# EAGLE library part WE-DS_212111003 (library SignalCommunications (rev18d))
WE-DS D-SUB-Filter, Solder Pin Straight Characteristics Standard type filtered with 1000 pF High attenuation: max. ≥ 40 dB @ 180 MHz Choice of UNC 4/40 or through hole Rated voltage: 100 VDC Rated current @ 20 ºC: 5 A Withstand voltage: 250 VRMS Insulation resistance: min. 1000 MΩ Operating temperature: –55 ºC to +125 ºC Applications Filtering of interfaces External connection to -printer -sensor -display Details see: http://katalog.we-online.de/en/pbs/Filter_gerade Created on 2015-05-04 2015 (C) Wurth Elektronik
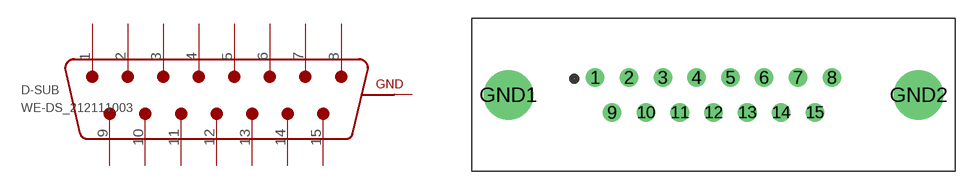
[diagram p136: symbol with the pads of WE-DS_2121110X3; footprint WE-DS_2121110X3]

Designator prefix D-SUB

## WE-DS_212111003 (WE-NUMBER: 212111003/15pins_male)  [WE-DS_2121110X3]
1  1  pas
2  2  pas
3  3  pas
4  4  pas
5  5  pas
6  6  pas
7  7  pas
8  8  pas
9  9  pas
10  10  pas
11  11  pas
12  12  pas
13  13  pas
14  14  pas
15  15  pas
GND1  GND  pas
GND2  GND  pas

## Footprint WE-DS_2121110X3 (pad centres in mm)
drill 1: 1 -9.6,1.42; 2 -6.86,1.42; 3 -4.11,1.42; 4 -1.37,1.42; 5 1.37,1.42; 6 4.11,1.42; 7 6.86,1.42; 8 9.6,1.42; 9 -8.23,-1.42; 10 -5.48,-1.42; 11 -2.74,-1.42; 12 0,-1.42; 13 2.74,-1.42; 14 5.48,-1.42; 15 8.23,-1.42
drill 3: GND1 -16.65,0; GND2 16.65,0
